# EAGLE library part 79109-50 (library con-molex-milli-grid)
RECEPTACAL
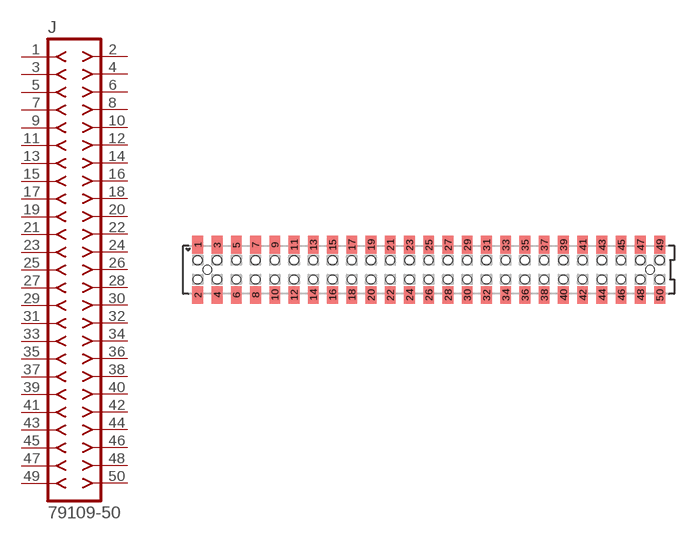
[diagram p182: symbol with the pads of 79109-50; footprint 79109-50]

Designator prefix J

## 79109-50  [79109-50]
1  1  pas
2  2  pas
3  3  pas
4  4  pas
5  5  pas
6  6  pas
7  7  pas
8  8  pas
9  9  pas
10  10  pas
11  11  pas
12  12  pas
13  13  pas
14  14  pas
15  15  pas
16  16  pas
17  17  pas
18  18  pas
19  19  pas
20  20  pas
21  21  pas
22  22  pas
23  23  pas
24  24  pas
25  25  pas
26  26  pas
27  27  pas
28  28  pas
29  29  pas
30  30  pas
31  31  pas
32  32  pas
33  33  pas
34  34  pas
35  35  pas
36  36  pas
37  37  pas
38  38  pas
39  39  pas
40  40  pas
41  41  pas
42  42  pas
43  43  pas
44  44  pas
45  45  pas
46  46  pas
47  47  pas
48  48  pas
49  49  pas
50  50  pas

## Footprint 79109-50 (pad centres in mm)
RECEPTACAL SMD Dual Row, Vertical, Pass-Thru
smd 1.12 x 1.83: 1 -24,2.6; 2 -24,-2.6; 3 -22,2.6; 4 -22,-2.6; 5 -20,2.6; 6 -20,-2.6; 7 -18,2.6; 8 -18,-2.6; 9 -16,2.6; 10 -16,-2.6; 11 -14,2.6; 12 -14,-2.6; 13 -12,2.6; 14 -12,-2.6; 15 -10,2.6; 16 -10,-2.6; 17 -8,2.6; 18 -8,-2.6; 19 -6,2.6; 20 -6,-2.6; 21 -4,2.6; 22 -4,-2.6; 23 -2,2.6; 24 -2,-2.6; 25 0,2.6; 26 0,-2.6; 27 2,2.6; 28 2,-2.6; 29 4,2.6; 30 4,-2.6; 31 6,2.6; 32 6,-2.6; 33 8,2.6; 34 8,-2.6; 35 10,2.6; 36 10,-2.6; 37 12,2.6; 38 12,-2.6; 39 14,2.6; 40 14,-2.6; 41 16,2.6; 42 16,-2.6; 43 18,2.6; 44 18,-2.6; 45 20,2.6; 46 20,-2.6; 47 22,2.6; 48 22,-2.6; 49 24,2.6; 50 24,-2.6
hole 0.914 at -23,0
hole 0.914 at -24,1
hole 0.914 at -24,-1
hole 0.914 at -22,-1
hole 0.914 at -22,1
hole 0.914 at -20,-1
hole 0.914 at -20,1
hole 0.914 at -18,1
hole 0.914 at -18,-1
hole 0.914 at -16,1
hole 0.914 at -16,-1
hole 0.914 at -14,1
hole 0.914 at -14,-1
hole 0.914 at -12,1
hole 0.914 at -12,-1
hole 0.914 at -10,-1
hole 0.914 at -10,1
hole 0.914 at -8,1
hole 0.914 at -8,-1
hole 0.914 at -6,1
hole 0.914 at -6,-1
hole 0.914 at -4,1
hole 0.914 at -4,-1
hole 0.914 at -2,-1
hole 0.914 at -2,1
hole 0.914 at 0,1
hole 0.914 at 2,1
hole 0.914 at 4,1
hole 0.914 at 0,-1
hole 0.914 at 2,-1
hole 0.914 at 4,-1
hole 0.914 at 6,-1
hole 0.914 at 8,-1
hole 0.914 at 10,-1
hole 0.914 at 12,-1
hole 0.914 at 14,-1
hole 0.914 at 6,1
hole 0.914 at 8,1
hole 0.914 at 10,1
hole 0.914 at 12,1
hole 0.914 at 14,1
hole 0.914 at 16,-1
hole 0.914 at 18,-1
hole 0.914 at 16,1
hole 0.914 at 18,1
hole 0.914 at 20,1
hole 0.914 at 22,1
hole 0.914 at 24,1
hole 0.914 at 20,-1
hole 0.914 at 22,-1
hole 0.914 at 24,-1
hole 0.914 at 23,0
